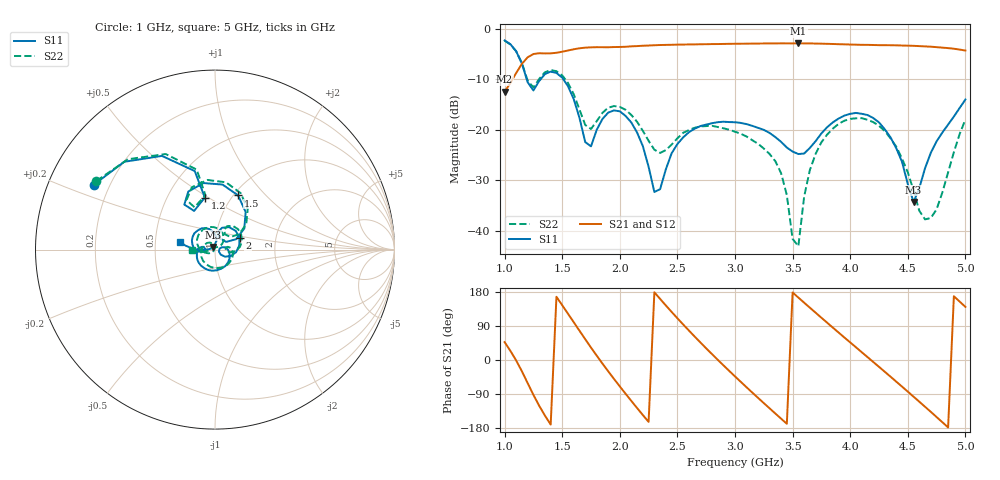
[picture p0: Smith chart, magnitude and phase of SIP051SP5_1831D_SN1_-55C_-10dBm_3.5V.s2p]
# GHz  S  dB  R  50
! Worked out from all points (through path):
!   81 points, 1 GHz to 5 GHz, reference 50 ohm
!   highest |S21| = -2.89 dB at 3.55 GHz (marker M1); lowest = -12.5 dB at 1 GHz (marker M2)
!   lowest |S11| = -34.3 dB at 4.55 GHz (marker M3), VSWR 1.04, Z = 48.8 + j1.43 ohm
!   |S11| at or under -10 dB: 1.192 GHz to 1.313 GHz (120.8 MHz wide, 9.65 % of centre); 1.51 GHz to end of sweep
!   |S22| runs from -43.1 to -2.3 dB; largest |S21 - S12| = 0.0022
!   S11 on the Smith chart (normalised r, x): 1 GHz: 0.14, +0.25; 1.2 GHz: 0.76, +0.48; 1.5 GHz: 1.05, +0.71; 2 GHz: 1.30, +0.18; 5 GHz: 0.67, +0.06
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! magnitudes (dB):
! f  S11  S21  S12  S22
! 1 GHz  -2.3  -12.5  -12.5  -2.3
! 1.2 GHz  -10.6  -5.7  -5.6  -10.3
! 1.5 GHz  -9.7  -4.5  -4.5  -9.2
! 1.7 GHz  -22.5  -3.7  -3.7  -19.1
! 2 GHz  -16.4  -3.6  -3.6  -15.5
! 2.15 GHz  -20.6  -3.4  -3.4  -18.4
! 2.3 GHz  -32.3  -3.3  -3.3  -24.0
! 2.35 GHz  -31.8  -3.2  -3.2  -24.6
! 2.45 GHz  -24.7  -3.2  -3.2  -22.9
! 2.6 GHz  -20.5  -3.1  -3.1  -20.1
! 3 GHz  -18.5  -3.0  -3.0  -20.4
! 3.35 GHz  -21.5  -2.9  -2.9  -26.2
! 3.45 GHz  -23.5  -2.9  -2.9  -32.9
! 3.5 GHz  -24.3  -2.9  -2.9  -41.6
! 3.55 GHz  -24.8  -2.9  -2.9  -43.1
! 3.6 GHz  -24.7  -2.9  -2.9  -33.3
! 3.7 GHz  -22.3  -2.9  -2.9  -24.8
! 4 GHz  -16.9  -3.1  -3.1  -17.9
! 4.35 GHz  -21.5  -3.3  -3.3  -21.7
! 4.55 GHz  -34.3  -3.4  -3.4  -32.1
! 4.7 GHz  -24.6  -3.6  -3.6  -37.5
! 5 GHz  -14.0  -4.3  -4.3  -18.0
